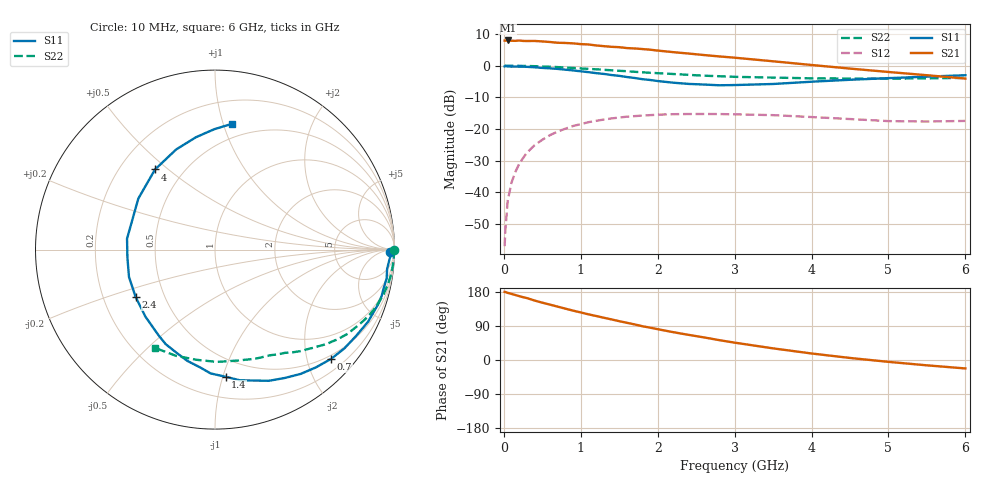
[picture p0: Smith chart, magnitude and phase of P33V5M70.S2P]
! SIEMENS Small Signal Semiconductors
! BFP181
! Si NPN RF Bipolar Junction Transistor in SOT143
! VCE = 3.5 V  IC = 0.7 mA
! Common Emitter S-Parameters:  March  1996
# GHz  S  MA  R  50
!  f  S11  S21  S12  S22
! GHz  MAG  ANG  MAG  ANG  MAG  ANG  MAG  ANG
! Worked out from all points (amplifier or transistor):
!   36 points, 10 MHz to 6 GHz, reference 50 ohm
!   highest |S21| = 8.0 dB at 50 MHz (marker M1)
!   |S21| within 3 dB of that: start of sweep to 1.929 GHz
!   unconditionally stable (mu >= 1): 3.553 GHz to end of sweep
!   at 250 MHz: K = 0.08, MSG = 18.5 dB, |S12| = -29.2 dB
!   at 1.4 GHz: K = 0.45, MSG = 11.3 dB, |S12| = -16.7 dB
!   at 6 GHz: K = 1.37, MAG = 3.1 dB, |S12| = -17.5 dB
!   S11 on the Smith chart (normalised r, x): 10 MHz: 62, -28; 700 MHz: 0.43, -2.46; 1.4 GHz: 0.36, -1.02; 2.4 GHz: 0.34, -0.25; 4 GHz: 0.35, +0.45; 6 GHz: 0.38, +1.07
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0.01  0.9737 -0.7  2.495 179.7  0.0014 93.0  0.9998 -0.1
0.02  0.9821 -1.4  2.486 179.5  0.0025 79.6  0.9983 -0.7
0.05  0.9748 -2.9  2.504 177.2  0.0073 90.2  0.997 -1.5
0.1  0.965 -6.4  2.477 174.4  0.0142 86.1  0.9973 -2.9
0.15  0.9697 -9.5  2.47 171.5  0.0209 83.3  0.995 -4.4
0.2  0.9644 -12.6  2.497 168.5  0.0281 81.3  0.9939 -6.0
0.3  0.9581 -18.7  2.453 163.4  0.0422 77.3  0.9888 -8.9
0.4  0.9427 -25.2  2.459 156.9  0.0552 72.7  0.9815 -11.8
0.5  0.9219 -31.4  2.417 151.3  0.0674 68.2  0.9723 -14.7
0.7  0.8885 -43.2  2.303 140.8  0.0908 60.6  0.9488 -20.1
0.9  0.8412 -55.4  2.252 130.3  0.1112 52.7  0.9206 -25.1
1.1  0.79 -67.7  2.164 120.5  0.1278 45.6  0.8898 -29.8
1.4  0.711 -85.2  1.986 107.1  0.1466 35.9  0.8457 -36.3
1.8  0.6121 -110.9  1.832 89.2  0.1624 25.4  0.7857 -43.4
2.2  0.5384 -136.1  1.637 73.5  0.171 16.0  0.7387 -50.0
2.4  0.515 -149.1  1.556 66.4  0.172 11.8  0.716 -53.1
3  0.4939 172.9  1.337 45.8  0.1701 1.5  0.6659 -62.0
3.5  0.5132 146.3  1.173 30.7  0.1651 -4.4  0.6482 -69.7
4  0.5576 126.8  1.025 17.2  0.1541 -8.7  0.6305 -78.8
4.5  0.5985 111.2  0.899 5.4  0.1432 -11.2  0.6258 -89.0
5.5  0.6706 90.4  0.706 -14.1  0.1309 -7.2  0.6305 -110.2
6  0.7061 82.5  0.625 -22.3  0.1338 -4.2  0.641 -121.2
